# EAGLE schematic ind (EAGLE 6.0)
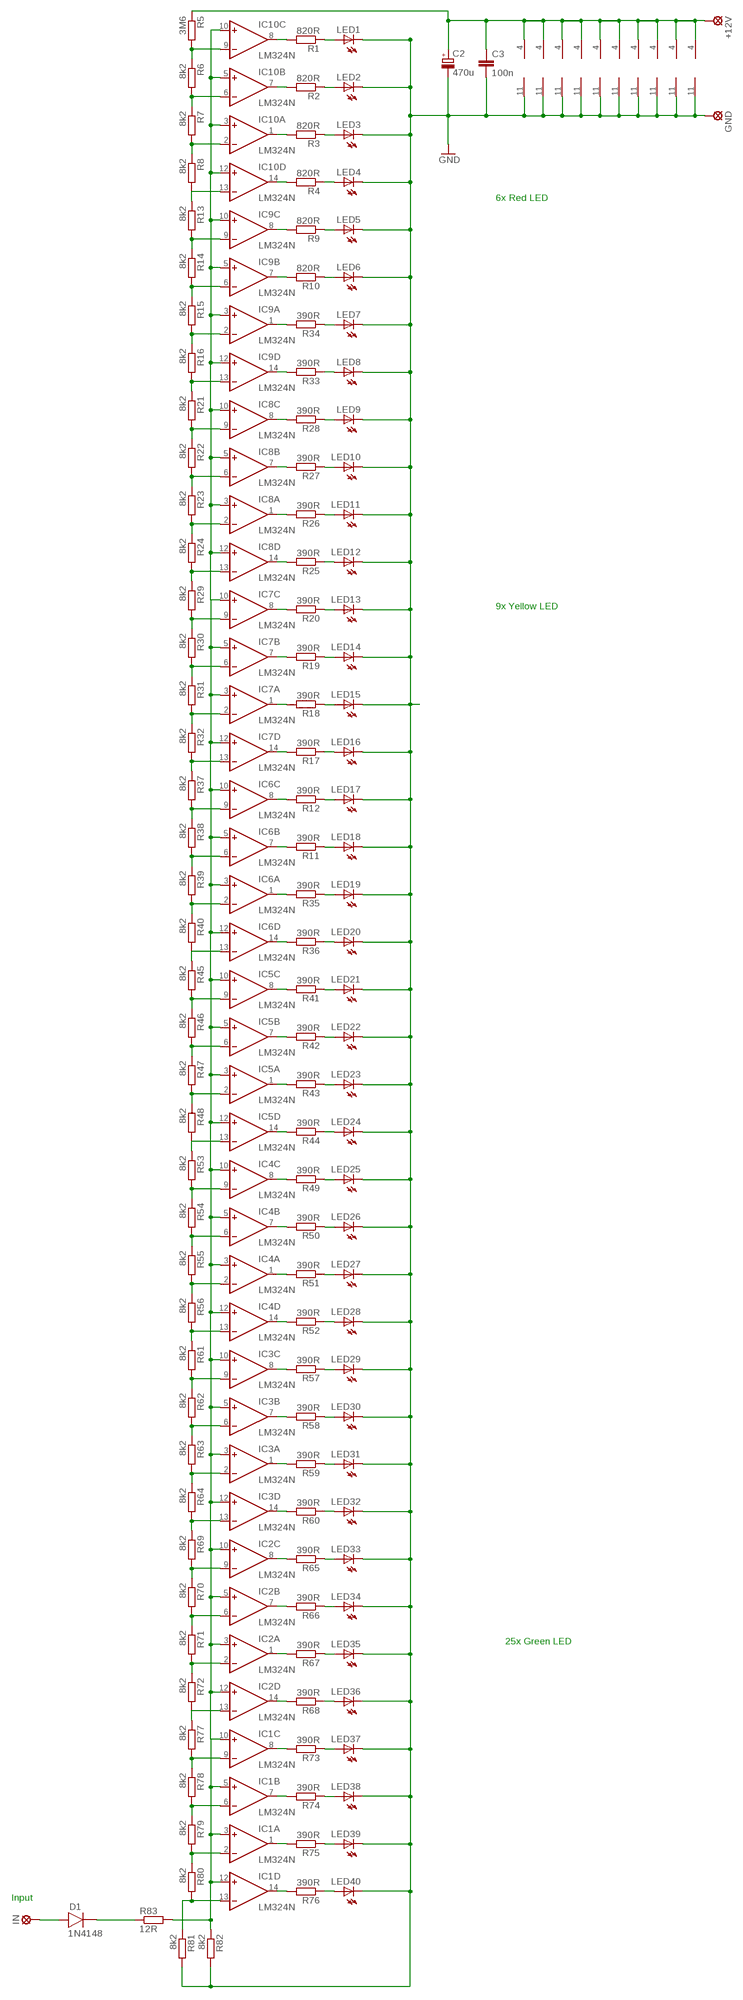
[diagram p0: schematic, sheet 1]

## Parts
+12V  LSP10  [LSP10]
C2  470u  CPOL-EUE2.5-7  [E2,5-7]
C3  100n  C-EU050-025X075  [C050-025X075]
D1  1N4148  [DO41]
GND  LSP10  [LSP10]
IC1  LM324N  [DIL14]
IC2  LM324N  [DIL14]
IC3  LM324N  [DIL14]
IC4  LM324N  [DIL14]
IC5  LM324N  [DIL14]
IC6  LM324N  [DIL14]
IC7  LM324N  [DIL14]
IC8  LM324N  [DIL14]
IC9  LM324N  [DIL14]
IC10  LM324N  [DIL14]
IN  LSP10  [LSP10]
LED1  LED5MM  [LED5MM]
LED2  LED5MM  [LED5MM]
LED3  LED5MM  [LED5MM]
LED4  LED5MM  [LED5MM]
LED5  LED5MM  [LED5MM]
LED6  LED5MM  [LED5MM]
LED7  LED5MM  [LED5MM]
LED8  LED5MM  [LED5MM]
LED9  LED5MM  [LED5MM]
LED10  LED5MM  [LED5MM]
LED11  LED5MM  [LED5MM]
LED12  LED5MM  [LED5MM]
LED13  LED5MM  [LED5MM]
LED14  LED5MM  [LED5MM]
LED15  LED5MM  [LED5MM]
LED16  LED5MM  [LED5MM]
LED17  LED5MM  [LED5MM]
LED18  LED5MM  [LED5MM]
LED19  LED5MM  [LED5MM]
LED20  LED5MM  [LED5MM]
LED21  LED5MM  [LED5MM]
LED22  LED5MM  [LED5MM]
LED23  LED5MM  [LED5MM]
LED24  LED5MM  [LED5MM]
LED25  LED5MM  [LED5MM]
LED26  LED5MM  [LED5MM]
LED27  LED5MM  [LED5MM]
LED28  LED5MM  [LED5MM]
LED29  LED5MM  [LED5MM]
LED30  LED5MM  [LED5MM]
LED31  LED5MM  [LED5MM]
LED32  LED5MM  [LED5MM]
LED33  LED5MM  [LED5MM]
LED34  LED5MM  [LED5MM]
LED35  LED5MM  [LED5MM]
LED36  LED5MM  [LED5MM]
LED37  LED5MM  [LED5MM]
LED38  LED5MM  [LED5MM]
LED39  LED5MM  [LED5MM]
LED40  LED5MM  [LED5MM]
R1  820R  R-EU_0207/10  [0207/10]
R2  820R  R-EU_0207/10  [0207/10]
R3  820R  R-EU_0207/10  [0207/10]
R4  820R  R-EU_0207/10  [0207/10]
R5  3M6  R-EU_0207/10  [0207/10]
R6  8k2  R-EU_0207/10  [0207/10]
R7  8k2  R-EU_0207/10  [0207/10]
R8  8k2  R-EU_0207/10  [0207/10]
R9  820R  R-EU_0207/10  [0207/10]
R10  820R  R-EU_0207/10  [0207/10]
R11  390R  R-EU_0207/10  [0207/10]
R12  390R  R-EU_0207/10  [0207/10]
R13  8k2  R-EU_0207/10  [0207/10]
R14  8k2  R-EU_0207/10  [0207/10]
R15  8k2  R-EU_0207/10  [0207/10]
R16  8k2  R-EU_0207/10  [0207/10]
R17  390R  R-EU_0207/10  [0207/10]
R18  390R  R-EU_0207/10  [0207/10]
R19  390R  R-EU_0207/10  [0207/10]
R20  390R  R-EU_0207/10  [0207/10]
R21  8k2  R-EU_0207/10  [0207/10]
R22  8k2  R-EU_0207/10  [0207/10]
R23  8k2  R-EU_0207/10  [0207/10]
R24  8k2  R-EU_0207/10  [0207/10]
R25  390R  R-EU_0207/10  [0207/10]
R26  390R  R-EU_0207/10  [0207/10]
R27  390R  R-EU_0207/10  [0207/10]
R28  390R  R-EU_0207/10  [0207/10]
R29  8k2  R-EU_0207/10  [0207/10]
R30  8k2  R-EU_0207/10  [0207/10]
R31  8k2  R-EU_0207/10  [0207/10]
R32  8k2  R-EU_0207/10  [0207/10]
R33  390R  R-EU_0207/10  [0207/10]
R34  390R  R-EU_0207/10  [0207/10]
R35  390R  R-EU_0207/10  [0207/10]
R36  390R  R-EU_0207/10  [0207/10]
R37  8k2  R-EU_0207/10  [0207/10]
R38  8k2  R-EU_0207/10  [0207/10]
R39  8k2  R-EU_0207/10  [0207/10]
R40  8k2  R-EU_0207/10  [0207/10]
R41  390R  R-EU_0207/10  [0207/10]
R42  390R  R-EU_0207/10  [0207/10]
R43  390R  R-EU_0207/10  [0207/10]
R44  390R  R-EU_0207/10  [0207/10]
R45  8k2  R-EU_0207/10  [0207/10]
R46  8k2  R-EU_0207/10  [0207/10]
R47  8k2  R-EU_0207/10  [0207/10]
R48  8k2  R-EU_0207/10  [0207/10]
R49  390R  R-EU_0207/10  [0207/10]
R50  390R  R-EU_0207/10  [0207/10]
R51  390R  R-EU_0207/10  [0207/10]
R52  390R  R-EU_0207/10  [0207/10]
R53  8k2  R-EU_0207/10  [0207/10]
R54  8k2  R-EU_0207/10  [0207/10]
R55  8k2  R-EU_0207/10  [0207/10]
R56  8k2  R-EU_0207/10  [0207/10]
R57  390R  R-EU_0207/10  [0207/10]
R58  390R  R-EU_0207/10  [0207/10]
R59  390R  R-EU_0207/10  [0207/10]
R60  390R  R-EU_0207/10  [0207/10]
R61  8k2  R-EU_0207/10  [0207/10]
R62  8k2  R-EU_0207/10  [0207/10]
R63  8k2  R-EU_0207/10  [0207/10]
R64  8k2  R-EU_0207/10  [0207/10]
R65  390R  R-EU_0207/10  [0207/10]
R66  390R  R-EU_0207/10  [0207/10]
R67  390R  R-EU_0207/10  [0207/10]
R68  390R  R-EU_0207/10  [0207/10]
R69  8k2  R-EU_0207/10  [0207/10]
R70  8k2  R-EU_0207/10  [0207/10]
R71  8k2  R-EU_0207/10  [0207/10]
R72  8k2  R-EU_0207/10  [0207/10]
R73  390R  R-EU_0207/10  [0207/10]
R74  390R  R-EU_0207/10  [0207/10]
R75  390R  R-EU_0207/10  [0207/10]
R76  390R  R-EU_0207/10  [0207/10]
R77  8k2  R-EU_0207/10  [0207/10]
R78  8k2  R-EU_0207/10  [0207/10]
R79  8k2  R-EU_0207/10  [0207/10]
R80  8k2  R-EU_0207/10  [0207/10]
R81  8k2  R-EU_0207/10  [0207/10]
R82  8k2  R-EU_0207/10  [0207/10]
R83  12R  R-EU_0207/10  [0207/10]

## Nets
GND: C2.- C3.2 GND.MP IC1.11(P:V-) IC2.11(P:V-) IC3.11(P:V-) IC4.11(P:V-) IC5.11(P:V-) IC6.11(P:V-) IC7.11(P:V-) IC8.11(P:V-) IC9.11(P:V-) IC10.11(P:V-) LED1.K(C) LED2.K(C) LED3.K(C) LED4.K(C) LED5.K(C) LED6.K(C) LED7.K(C) LED8.K(C) LED9.K(C) LED10.K(C) LED11.K(C) LED12.K(C) LED13.K(C) LED14.K(C) LED15.K(C) LED16.K(C) LED17.K(C) LED18.K(C) LED19.K(C) LED20.K(C) LED21.K(C) LED22.K(C) LED23.K(C) LED24.K(C) LED25.K(C) LED26.K(C) LED27.K(C) LED28.K(C) LED29.K(C) LED30.K(C) LED31.K(C) LED32.K(C) LED33.K(C) LED34.K(C) LED35.K(C) LED36.K(C) LED37.K(C) LED38.K(C) LED39.K(C) LED40.K(C) R81.2 R82.2
N$1: LED1.A R1.1
N$2: LED2.A R2.1
N$3: LED3.A R3.1
N$4: IC10.14(D:OUT) R4.2
N$5: IC10.8(C:OUT) R1.2
N$6: IC10.7(B:OUT) R2.2
N$7: IC10.1(A:OUT) R3.2
N$8: LED4.A R4.1
N$9: LED17.A R12.1
N$10: IC10.9(C:-IN) R5.2 R6.1
N$11: IC10.6(B:-IN) R6.2 R7.1
N$12: IC10.2(A:-IN) R7.2 R8.1
N$13: IC10.13(D:-IN) R8.2 R13.1
N$14: LED5.A R9.1
N$15: LED6.A R10.1
N$16: LED7.A R34.1
N$17: IC9.14(D:OUT) R33.2
N$18: IC9.8(C:OUT) R9.2
N$19: IC9.7(B:OUT) R10.2
N$20: IC9.1(A:OUT) R34.2
N$21: LED8.A R33.1
N$22: LED18.A R11.1
N$23: IC9.9(C:-IN) R13.2 R14.1
N$24: IC9.6(B:-IN) R14.2 R15.1
N$25: IC9.2(A:-IN) R15.2 R16.1
N$26: IC9.13(D:-IN) R16.2 R21.1
N$27: LED9.A R28.1
N$28: LED10.A R27.1
N$29: LED11.A R26.1
N$30: IC8.14(D:OUT) R25.2
N$31: IC8.8(C:OUT) R28.2
N$32: IC8.7(B:OUT) R27.2
N$33: IC8.1(A:OUT) R26.2
N$34: LED12.A R25.1
N$35: IC8.9(C:-IN) R21.2 R22.1
N$36: IC8.6(B:-IN) R22.2 R23.1
N$37: IC8.2(A:-IN) R23.2 R24.1
N$38: IC8.13(D:-IN) R24.2 R29.1
N$39: LED13.A R20.1
N$40: LED14.A R19.1
N$41: LED15.A R18.1
N$42: IC7.14(D:OUT) R17.2
N$43: IC7.8(C:OUT) R20.2
N$44: IC7.7(B:OUT) R19.2
N$45: IC7.1(A:OUT) R18.2
N$46: LED16.A R17.1
N$47: D1.A IN.MP
N$48: IC7.9(C:-IN) R29.2 R30.1
N$49: IC7.6(B:-IN) R30.2 R31.1
N$50: IC7.2(A:-IN) R31.2 R32.1
N$51: IC7.13(D:-IN) R32.2 R37.1
N$52: LED19.A R35.1
N$53: IC6.14(D:OUT) R36.2
N$54: IC6.8(C:OUT) R12.2
N$55: IC6.7(B:OUT) R11.2
N$56: IC6.1(A:OUT) R35.2
N$57: LED20.A R36.1
N$58: IC6.9(C:-IN) R37.2 R38.1
N$59: IC6.6(B:-IN) R38.2 R39.1
N$60: IC6.2(A:-IN) R39.2 R40.1
N$61: IC6.13(D:-IN) R40.2 R45.1
N$62: LED21.A R41.1
N$63: LED22.A R42.1
N$64: LED23.A R43.1
N$65: IC5.14(D:OUT) R44.2
N$66: IC5.8(C:OUT) R41.2
N$67: IC5.7(B:OUT) R42.2
N$68: IC5.1(A:OUT) R43.2
N$69: LED24.A R44.1
N$70: IC5.9(C:-IN) R45.2 R46.1
N$71: IC5.6(B:-IN) R46.2 R47.1
N$72: IC5.2(A:-IN) R47.2 R48.1
N$73: IC5.13(D:-IN) R48.2 R53.1
N$74: LED25.A R49.1
N$75: LED26.A R50.1
N$76: LED27.A R51.1
N$77: IC4.14(D:OUT) R52.2
N$78: IC4.8(C:OUT) R49.2
N$79: IC4.7(B:OUT) R50.2
N$80: IC4.1(A:OUT) R51.2
N$81: LED28.A R52.1
N$82: IC4.9(C:-IN) R53.2 R54.1
N$83: IC4.6(B:-IN) R54.2 R55.1
N$84: IC4.2(A:-IN) R55.2 R56.1
N$85: IC4.13(D:-IN) R56.2 R61.1
N$86: LED29.A R57.1
N$87: LED30.A R58.1
N$88: LED31.A R59.1
N$89: IC3.14(D:OUT) R60.2
N$90: IC3.8(C:OUT) R57.2
N$91: IC3.7(B:OUT) R58.2
N$92: IC3.1(A:OUT) R59.2
N$93: LED32.A R60.1
N$95: IC3.9(C:-IN) R61.2 R62.1
N$96: IC3.6(B:-IN) R62.2 R63.1
N$97: IC3.2(A:-IN) R63.2 R64.1
N$98: IC3.13(D:-IN) R64.2 R69.1
N$99: LED33.A R65.1
N$100: LED34.A R66.1
N$101: LED35.A R67.1
N$102: IC2.14(D:OUT) R68.2
N$103: IC2.8(C:OUT) R65.2
N$104: IC2.7(B:OUT) R66.2
N$105: IC2.1(A:OUT) R67.2
N$106: LED36.A R68.1
N$107: IC2.9(C:-IN) R69.2 R70.1
N$108: IC2.6(B:-IN) R70.2 R71.1
N$109: IC2.2(A:-IN) R71.2 R72.1
N$110: IC2.13(D:-IN) R72.2 R77.1
N$111: LED37.A R73.1
N$112: LED38.A R74.1
N$113: LED39.A R75.1
N$114: IC1.14(D:OUT) R76.2
N$115: IC1.8(C:OUT) R73.2
N$116: IC1.7(B:OUT) R74.2
N$117: IC1.1(A:OUT) R75.2
N$118: LED40.A R76.1
N$119: +12V.MP C2.+ C3.1 IC1.4(P:V+) IC2.4(P:V+) IC3.4(P:V+) IC4.4(P:V+) IC5.4(P:V+) IC6.4(P:V+) IC7.4(P:V+) IC8.4(P:V+) IC9.4(P:V+) IC10.4(P:V+) R5.1
N$120: IC1.9(C:-IN) R77.2 R78.1
N$121: IC1.6(B:-IN) R78.2 R79.1
N$122: IC1.2(A:-IN) R79.2 R80.1
N$123: IC1.13(D:-IN) R80.2 R81.1
N$124: IC1.3(A:+IN) IC1.5(B:+IN) IC1.10(C:+IN) IC1.12(D:+IN) IC2.3(A:+IN) IC2.5(B:+IN) IC2.10(C:+IN) IC2.12(D:+IN) IC3.3(A:+IN) IC3.5(B:+IN) IC3.10(C:+IN) IC3.12(D:+IN) IC4.3(A:+IN) IC4.5(B:+IN) IC4.10(C:+IN) IC4.12(D:+IN) IC5.3(A:+IN) IC5.5(B:+IN) IC5.10(C:+IN) IC5.12(D:+IN) IC6.3(A:+IN) IC6.5(B:+IN) IC6.10(C:+IN) IC6.12(D:+IN) IC7.3(A:+IN) IC7.5(B:+IN) IC7.10(C:+IN) IC7.12(D:+IN) IC8.3(A:+IN) IC8.5(B:+IN) IC8.10(C:+IN) IC8.12(D:+IN) IC9.3(A:+IN) IC9.5(B:+IN) IC9.10(C:+IN) IC9.12(D:+IN) IC10.3(A:+IN) IC10.5(B:+IN) IC10.10(C:+IN) IC10.12(D:+IN) R82.1 R83.2
N$125: D1.K R83.1

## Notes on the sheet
- 6x Red LED
- 9x Yellow LED
- 25x Green LED
- Input

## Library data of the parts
+12V GND IN = solpad:LSP10: SOLDER PAD
C2 = rcl:CPOL-EU: POLARIZED CAPACITOR, European symbol
C3 = rcl:C-EU: CAPACITOR, European symbol
D1 = GM99:1N4148
IC1-IC10 = linear:LM324: OP AMP
LED1-LED40 = led:LED: LED
R1-R83 = rcl:R-EU_: RESISTOR, European symbol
